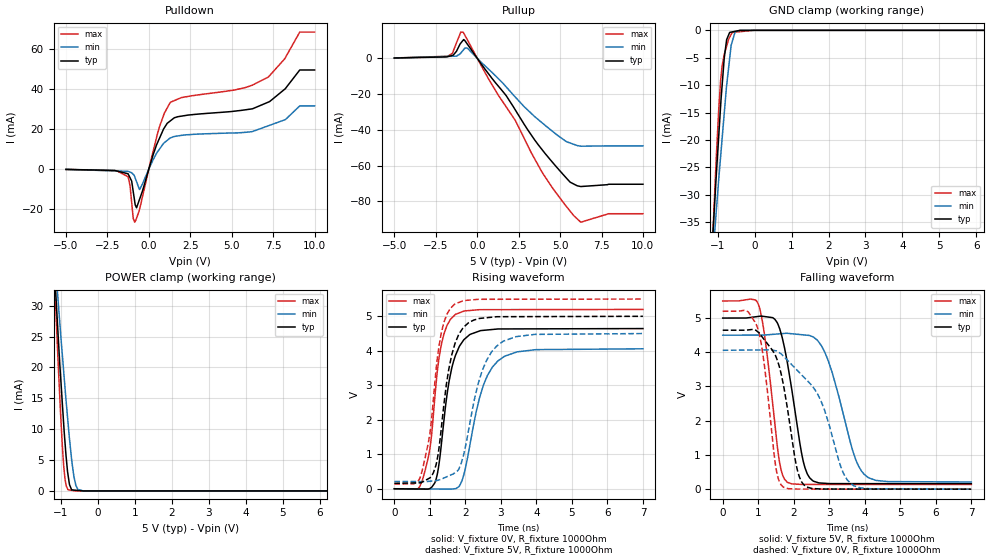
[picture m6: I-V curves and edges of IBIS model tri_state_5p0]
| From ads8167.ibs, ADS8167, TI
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|   tri_state_5p0 Model
[Model]   tri_state_5p0
Model_type   3-state
Polarity   Non-Inverting
Vmeas = 2.5
Vref = 0
Cref = 2pF
Rref = 100000
|   typ   min   max
C_comp   1.1130E-12F   1.0764E-12F   1.1266E-12F
|  Where Nom  PVT is Nominal Process, 5V,   27C
|   Fast PVT is Strong Process,  5.5V, -40C
|   Slow PVT is Weak Process,   4.5V, 125C
[Voltage Range]   5   4.5   5.5
|Junction Temperature
[Temperature Range]   27   125   -40
[Pullup Reference]   5   4.5   5.5
[Pulldown Reference]   0   0   0
[Power Clamp Reference]   5   4.5   5.5
[GND Clamp Reference]   0   0   0
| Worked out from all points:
|   slope of the pulldown table from 0 to 0.75 V, typ, clamps not added: 43 ohm
|   slope of the pullup table from 0 to 0.75 V, typ, clamps not added: 78.9 ohm
|   GND clamp passes 1 mA (typ) near -0.71 V on its own axis
|   POWER clamp passes 1 mA (typ) near -0.77 V on its own axis
|   falling waveform, V_fixture 5V, R_fixture 1000Ohm: 20-80 % time 449ps typ, 671ps min, 356ps max; typ from 5 V to 0.158 V
|   rising waveform, V_fixture 0V, R_fixture 1000Ohm: 20-80 % time 389ps typ, 562ps min, 338ps max; typ from 0 V to 4.64 V
|   rising waveform, V_fixture 5V, R_fixture 1000Ohm: 20-80 % time 407ps typ, 593ps min, 375ps max; typ from 0.158 V to 5 V
|   falling waveform, V_fixture 0V, R_fixture 1000Ohm: 20-80 % time 475ps typ, 966ps min, 346ps max; typ from 4.64 V to 0 V
[Pulldown]
|   Voltage   I(typ)   I(min)   I(max)
-5V       -186.4uA   -146.8uA   -188.1uA
-1.25V    -2.374mA   -1.157mA   -3.876mA
-1.036V   -6.028mA   -1.855mA   -16.65mA
-858.2mV  -15.92mA   -3.69mA    -26.62mA
-741mV    -19.4mA    -6.327mA   -24.58mA
-543.6mV  -14.77mA   -10.1mA    -19.59mA
546.1mV   13.61mA    8.871mA    18.44mA
1.321V    24.29mA    15.66mA    33.52mA
6.25V     30.17mA    18.78mA    42.02mA
8.202V    40.02mA    24.66mA    55.26mA
9.106V    49.62mA    31.63mA    68.6mA
10V       49.62mA    31.63mA    68.6mA
[GND Clamp]
|   Voltage   I(typ)   I(min)   I(max)
-5V       -547.1mA   -430.6mA   -696mA
-1.25V    -51.51mA   -52.28mA   -55.31mA
-1.037V   -26.38mA   -32.95mA   -23.13mA
-971mV    -19.28mA   -27.19mA   -14.46mA
-878.3mV  -9.952mA   -19.68mA   -6.405mA
-821.2mV  -4.995mA   -15.1mA    -4.377mA
-756.7mV  -1.693mA   -10.04mA   -2.87mA
-675mV    -379.9uA   -5.118mA   -1.272mA
-635.7mV  -327.1uA   -2.756mA   -755.2uA
-527.4mV  -181.3uA   -262.8uA   -324.5uA
-393mV    -429.7nA   -6.203uA   -241.8uA
10V       0A         0A         0A
[Pullup]
|   Voltage   I(typ)   I(min)   I(max)
-5V       134.2uA    105.7uA    145.7uA
-1.776V   905.6uA    1.024mA    1.105mA
-1.495V   1.554mA    1.104mA    2.74mA
-988.5mV  8.464mA    2.917mA    14.6mA
-854.7mV  10.04mA    4.411mA    14.62mA
-573.3mV  7.604mA    5.466mA    9.963mA
2.289V    -28.75mA   -21.62mA   -34.61mA
3.892V    -50.82mA   -35.91mA   -63.33mA
5.82V     -70.28mA   -48.09mA   -87.94mA
6.25V     -71.72mA   -49.17mA   -91.64mA
7.932V    -70.43mA   -48.98mA   -86.91mA
10V       -70.43mA   -48.98mA   -86.91mA
[POWER Clamp]
|   Voltage   I(typ)   I(min)   I(max)
-5V       483mA      386.8mA    606.2mA
-1.25V    43.72mA    44.95mA    44.68mA
-1.122V   30.22mA    34.47mA    27.24mA
-1.073V   24.99mA    30.59mA    20.48mA
-1.012V   18.84mA    25.83mA    12.85mA
-925.7mV  10.87mA    19.39mA    4.118mA
-890.4mV  7.924mA    16.79mA    1.962mA
-806.9mV  2.572mA    11.01mA    182.2uA
-706.8mV  166.6uA    4.89mA     90.98uA
-597.7mV  108.7uA    928.8uA    154.6nA
-393mV    14.02nA    3.586uA    101.7nA
10V       0A         0A         0A
[Ramp]
R_load = 1000
|   typ   min   max
dV/dt_r   2.78666/3.88336e-10   2.43472/5.59556e-10   3.1193/3.38049e-10
dV/dt_f   2.90514/4.47583e-10   2.5742/6.68213e-10   3.2182/3.55238e-10
[Falling Waveform]
V_fixture = 5V
V_fixture_min = 4.5V
V_fixture_max = 5.5V
R_fixture = 1000Ohm
C_fixture = 0F
|   Time   V(typ)   V(min)   V(max)
0s        5V         4.5V       5.5V
1.011ns   5.049V     4.501V     5.382V
1.23ns    5.037V     4.508V     4.1V
1.589ns   4.729V     4.538V     861mV
1.809ns   3.763V     4.555V     211.7mV
2.258ns   860.7mV    4.51V      138.9mV
2.538ns   244.4mV    4.453V     138.7mV
2.96ns    165.6mV    3.784V     138.5mV
3.99ns    161.4mV    426.3mV    137.9mV
7ns       158.1mV    209.6mV    136.3mV
[Rising Waveform]
V_fixture = 0V
V_fixture_min = 0V
V_fixture_max = 0V
R_fixture = 1000Ohm
C_fixture = 0F
|   Time   V(typ)   V(min)   V(max)
0s        7.976uV    152.8uV    -146.6nV
775.3ps   -8.611mV   -4.784mV   201.9mV
1.011ns   15.64mV    -6.288mV   1.234V
1.142ns   178mV      -7.12mV    2.671V
1.33ns    1.341V     -8.315mV   4.208V
1.709ns   3.83V      2.222mV    5.046V
1.942ns   4.297V     351.6mV    5.144V
2.502ns   4.593V     2.983V     5.193V
2.912ns   4.633V     3.701V     5.193V
7ns       4.644V     4.058V     5.199V
[Rising Waveform]
V_fixture = 5V
V_fixture_min = 4.5V
V_fixture_max = 5.5V
R_fixture = 1000Ohm
C_fixture = 0F
|   Time   V(typ)   V(min)   V(max)
0s        158.1mV    209.6mV    136.3mV
706.2ps   171.7mV    208.5mV    278.2mV
964ps     293.6mV    214.7mV    1.369V
1.103ns   475.5mV    226mV      2.638V
1.33ns    1.822V     281.3mV    4.551V
1.689ns   4.143V     452.5mV    5.344V
1.952ns   4.685V     986.1mV    5.455V
2.482ns   4.947V     3.443V     5.494V
3.05ns    4.989V     4.267V     5.494V
7ns       5V         4.5V       5.5V
[Falling Waveform]
|Gnd
V_fixture = 0V
V_fixture_min = 0V
V_fixture_max = 0V
R_fixture = 1000Ohm
C_fixture = 0F
|   Time   V(typ)   V(min)   V(max)
0s        4.644V     4.058V     5.199V
977.2ps   4.607V     4.067V     4.729V
1.171ns   4.368V     4.069V     3.641V
1.499ns   3.872V     4.043V     621.9mV
1.699ns   3.104V     3.899V     67.49mV
2.098ns   577.1mV    3.473V     2.355mV
2.358ns   67.2mV     3.195V     2.23mV
2.752ns   5.725mV    2.614V     2.041mV
3.68ns    2.84mV     106.5mV    1.595mV
7ns       7.818uV    152.7uV    -37.25nV
